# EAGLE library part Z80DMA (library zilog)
Z80 FAMILY DEVICE
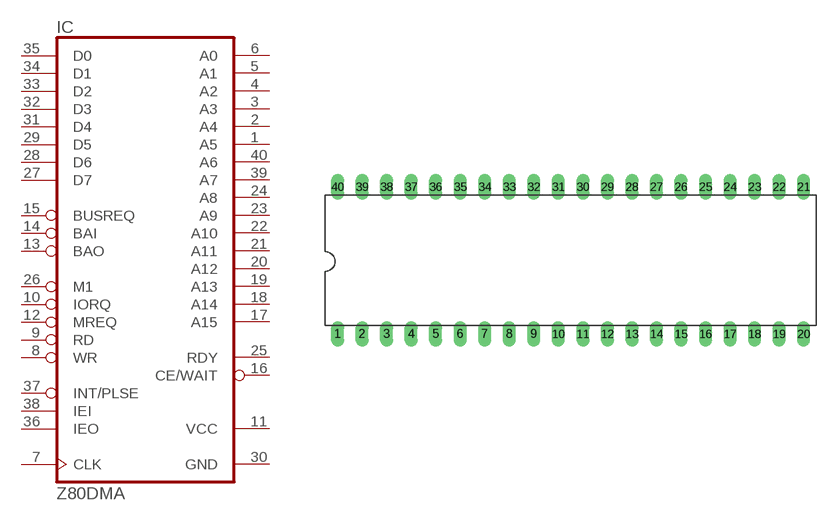
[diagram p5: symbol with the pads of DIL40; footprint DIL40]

Designator prefix IC

## Z80DMA  [DIL40]
1  A5  out
2  A4  out
3  A3  out
4  A2  out
5  A1  out
6  A0  out
7  CLK  in
8  WR
9  RD
10  IORQ
11  VCC  pwr
12  MREQ  out
13  BAO  out
14  BAI  in
15  BUSREQ
16  CE/WAIT  in
17  A15  out
18  A14  out
19  A13  out
20  A12  out
21  A11  out
22  A10  out
23  A9  out
24  A8  out
25  RDY  in
26  M1  in
27  D7
28  D6
29  D5
30  GND  pwr
31  D4
32  D3
33  D2
34  D1
35  D0
36  IEO  out
37  INT/PLSE  oc
38  IEI  in
39  A7  out
40  A6  out

## Footprint DIL40 (pad centres in mm)
Dual In Line Package
drill 0.813 long: 1 -24.13,-7.62; 2 -21.59,-7.62; 3 -19.05,-7.62; 4 -16.51,-7.62; 5 -13.97,-7.62; 6 -11.43,-7.62; 7 -8.89,-7.62; 8 -6.35,-7.62; 9 -3.81,-7.62; 10 -1.27,-7.62; 11 1.27,-7.62; 12 3.81,-7.62; 13 6.35,-7.62; 14 8.89,-7.62; 15 11.43,-7.62; 16 13.97,-7.62; 17 16.51,-7.62; 18 19.05,-7.62; 19 21.59,-7.62; 20 24.13,-7.62; 21 24.13,7.62; 22 21.59,7.62; 23 19.05,7.62; 24 16.51,7.62; 25 13.97,7.62; 26 11.43,7.62; 27 8.89,7.62; 28 6.35,7.62; 29 3.81,7.62; 30 1.27,7.62; 31 -1.27,7.62; 32 -3.81,7.62; 33 -6.35,7.62; 34 -8.89,7.62; 35 -11.43,7.62; 36 -13.97,7.62; 37 -16.51,7.62; 38 -19.05,7.62; 39 -21.59,7.62; 40 -24.13,7.62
